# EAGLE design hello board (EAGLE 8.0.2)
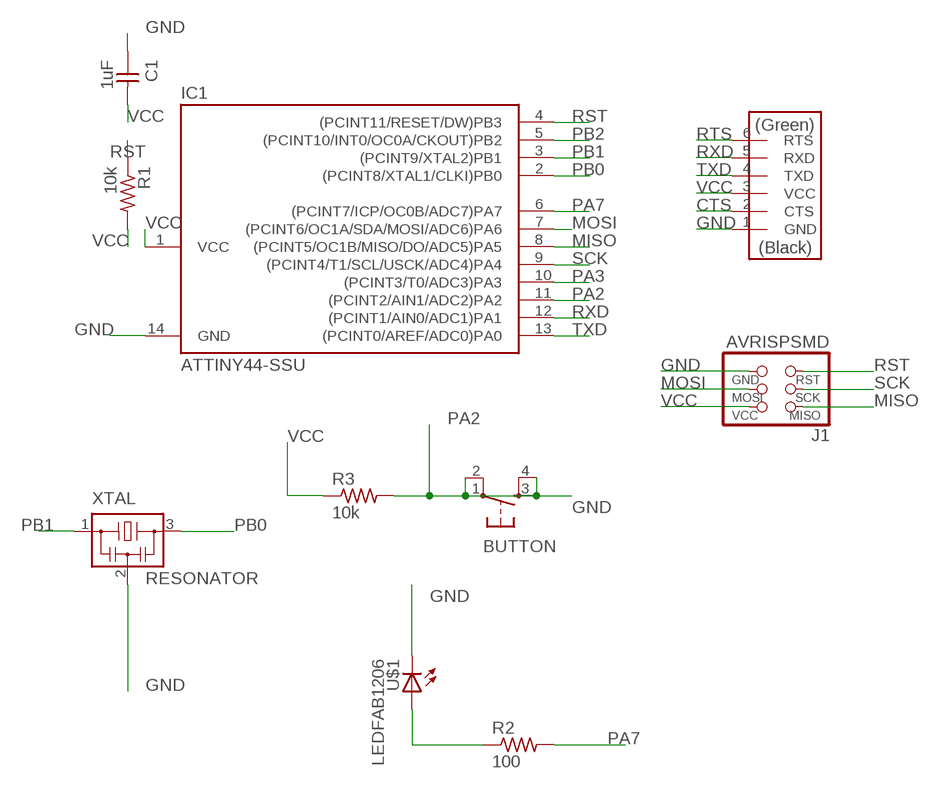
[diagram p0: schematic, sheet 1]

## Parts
BUTTON  6MM_SWITCH6MM_SWITCH  [6MM_SWITCH]
C1  1uF  CAP-UNPOLARIZEDFAB  [C1206FAB]
IC1  ATTINY44-SSU  [SOIC14]
J1  AVRISPSMD  [2X03SMD]
R1  10k  RES-US1206W  [R1206W]
R2  100  RES-US1206FAB  [R1206FAB]
R3  10k  RES-US1206FAB  [R1206FAB]
U$1  LEDFAB1206  [LED1206FAB]
U$2  FTDI-SMD-HEADER  [1X06SMD]
XTAL  RESONATOR  [EFOBM]

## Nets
CTS: U$2.2(CTS)
GND: BUTTON.1(P) BUTTON.2(P1) C1.1 IC1.14(GND) J1.6(GND) U$1.2(C) U$2.1(GND) XTAL.2
MISO: IC1.8((PCINT5/OC1B/MISO/DO/ADC5)PA5) J1.1(MISO)
MOSI: IC1.7((PCINT6/OC1A/SDA/MOSI/ADC6)PA6) J1.4(MOSI)
N$1: R2.1 U$1.1(A)
PA2: BUTTON.3(S) BUTTON.4(S1) IC1.11((PCINT2/AIN1/ADC2)PA2) R3.2
PA3: IC1.10((PCINT3/T0/ADC3)PA3)
PA7: IC1.6((PCINT7/ICP/OC0B/ADC7)PA7) R2.2
PB0: IC1.2((PCINT8/XTAL1/CLKI)PB0) XTAL.3
PB1: IC1.3((PCINT9/XTAL2)PB1) XTAL.1
PB2: IC1.5((PCINT10/INT0/OC0A/CKOUT)PB2)
RST: IC1.4((PCINT11/RESET/DW)PB3) J1.5(RST) R1.1
RTS: U$2.6(RTS)
RXD: IC1.12((PCINT1/AIN0/ADC1)PA1) U$2.5(RXD)
SCK: IC1.9((PCINT4/T1/SCL/USCK/ADC4)PA4) J1.3(SCK)
TXD: IC1.13((PCINT0/AREF/ADC0)PA0) U$2.4(TXD)
VCC: C1.2 IC1.1(VCC) J1.2(VCC) R1.2 R3.1 U$2.3(VCC)

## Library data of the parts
BUTTON = fab:6MM_SWITCH: OMRON SWITCH
C1 = fab:CAP-UNPOLARIZED
IC1 = fab:ATTINY44
J1 = fab:AVRISP
R1-R3 = fab:RES-US: Resistor (US Symbol)
U$1 = fab:LED: LED
U$2 = fab:FTDI-SMD-HEADER
XTAL = fab:RESONATOR

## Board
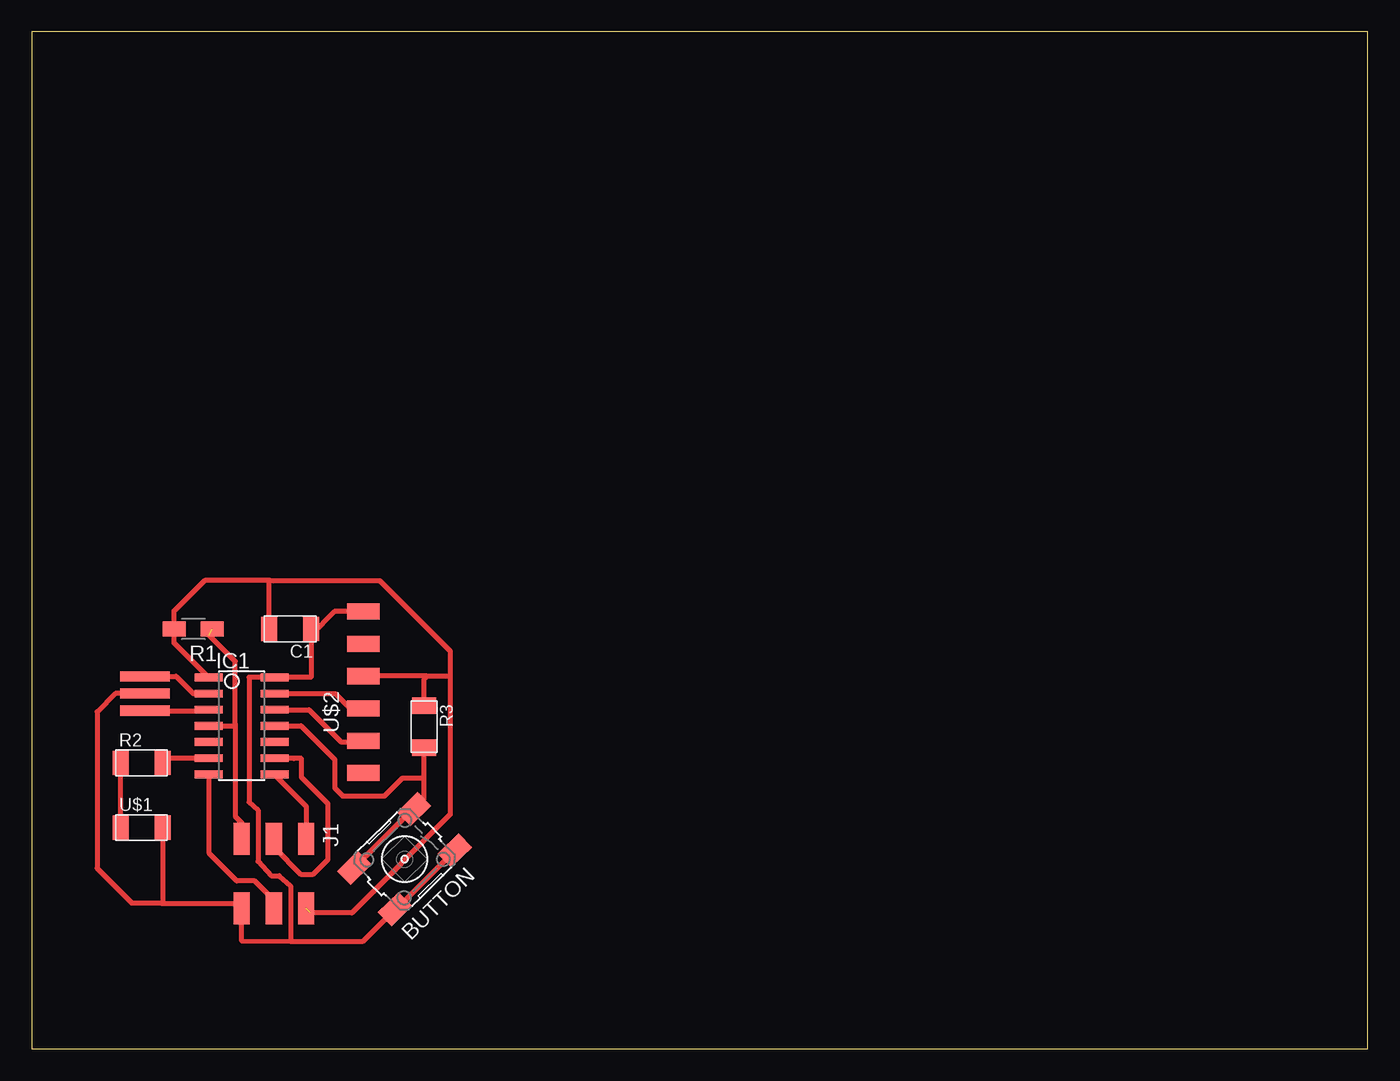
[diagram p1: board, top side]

Size 105.08 x 80 mm. Coordinates in mm from the lower left corner, seen from the top.
Outline: 0,0 105.08,0 105.08,80 0,80 0,0
Copper layers (1*16): Top 0.035mm / dielectric 1.5mm / Bottom 0.035mm
Design rules "default *": minimum track width 10mil, minimum drill 24mil, track to track 16mil, track to pad 16mil, pad to pad 16mil, via to via 16mil, smd to smd 16mil, copper to edge 40mil, drill to drill 8mil, minimum pad ring 10mil, minimum via ring 8mil, stop-mask expansion 4mil, vias tented up to drill 0mil, thermal gap 10mil

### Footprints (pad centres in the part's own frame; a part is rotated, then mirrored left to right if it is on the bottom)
6MM_SWITCH = smd 2.286 x 1.524: 1 -3.302,2.286; 2 3.302,2.286; 3 -3.302,-2.286; 4 3.302,-2.286
C1206FAB = smd 1.27 x 1.905: 1 -1.651,0; 2 1.651,0
SOIC14 = smd 0.61 x 2.21: 1 -3.81,-2.603; 2 -2.54,-2.603; 3 -1.27,-2.603; 4 0,-2.603; 5 1.27,-2.603; 6 2.54,-2.603; 7 3.81,-2.603; 8 3.81,2.603; 9 2.54,2.603; 10 1.27,2.603; 11 0,2.603; 12 -1.27,2.603; 13 -2.54,2.603; 14 -3.81,2.603
2X03SMD = smd 2.54 x 1.27: 1 -2.54,2.54; 2 2.92,2.54; 3 -2.54,0; 4 2.92,0; 5 -2.54,-2.54; 6 2.92,-2.54
R1206W = smd 1.8 x 1.2: 1 -1.499,0; 2 1.499,0
R1206FAB = smd 1.27 x 1.905: 1 -1.651,0; 2 1.651,0
LED1206FAB = smd 1.27 x 1.905: 1 -1.651,0; 2 1.651,0
1X06SMD = smd 2.54 x 1.27: 1 0,6.35; 2 0,3.81; 3 0,1.27; 4 0,-1.27; 5 0,-3.81; 6 0,-6.35
EFOBM = smd 0.8 x 3.9: 1 -1.35,0; 2 0,0; 3 1.35,0

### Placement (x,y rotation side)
BUTTON  29.32,14.92 224.5 top
C1  20.32,33.02 180 top
IC1  16.51,25.4 270 top
J1  19.05,13.97 270 top
R1  12.7,33.02 180 top
R2  8.64,22.48 0 top
R3  30.86,25.33 270 top
U$1  8.64,17.4 0 top
U$2  26.08,28.04 0 top
XTAL  8.89,27.94 90 top

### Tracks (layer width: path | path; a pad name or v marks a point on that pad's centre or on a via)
GND
  Top 0.406: 21.59,33.02 C1.1 21.97,32.56 | J1.6 16.51,11.43 | XTAL.2 6.57,27.94 5.13,26.5 5.13,14.2 7.88,11.45 10.18,11.45 | 10.18,11.45 16.11,11.45 J1.6 | U$1.2 10.29,11.56 10.18,11.45 | 20.32,8.46 16.52,8.48 J1.6 | 26.06,34.4 U$2.1 23.8,34.39 21.97,32.56 | 19.16,29.16 IC1.14 | 21.97,32.56 21.97,29.21 IC1.14 | IC1.14 17.08,29.21 17.08,19.42 17.8,18.77 17.8,14.73 18.84,13.62 19.46,13.62 20.34,12.82 20.34,8.52 20.32,8.46 | 20.32,8.46 26.06,8.46 BUTTON.2 28.65,10.97 BUTTON.1
MISO
  Top 0.406: IC1.8 19.11,21.53 21.59,19.05 J1.1
MOSI
  Top 0.406: 13.97,21.59 IC1.7 13.97,21.53 13.97,15.37 16.13,13.21 17.53,13.21 19.05,11.68 J1.4
N$1
  Top 0.406: U$1.1 R2.1
PA2
  Top 0.406: IC1.11 21.17,25.4 23.83,22.75 23.83,20.5 24.45,19.89 27.74,19.89 29.16,21.3 30.81,21.3 | 30.81,21.3 30.84,21.34 30.84,23.66 R3.2 | 30.81,21.3 30.81,19.6 BUTTON.3 29.99,18.86 BUTTON.4
PA7
  Top 0.406: IC1.6 10.67,22.86 R2.2
PB0
  Top 0.406: XTAL.3 11.35,29.29 12.7,27.94 IC1.2
PB1
  Top 0.406: XTAL.1 13.83,26.59 IC1.3
RST  (1 unrouted)
  Top 0.406: J1.5 16.51,17.78 16,18.29 16,25.53 | 16,25.53 16,30.48 13.97,32.51 | IC1.4 15.88,25.4 16,25.53
RXD
  Top 0.406: IC1.12 21.8,26.67 24.33,24.15 25.99,24.15 U$2.5
SCK
  Top 0.406: IC1.9 20.59,22.86 20.62,22.83 21.21,22.83 21.21,21.36 23.3,19.28 23.3,14.88 22.14,13.73 21.15,13.73 19.05,15.83 J1.3
TXD
  Top 0.406: IC1.13 23.87,27.94 25.03,26.77 U$2.4
VCC  (1 unrouted)
  Top 0.406: IC1.1 11.2,31.92 R1.2 11.2,34.45 13.59,36.83 18.78,36.83 | 32.91,29.22 32.91,31.28 27.37,36.83 18.78,36.83 | J1.2 21.7,10.95 | 31.09,29.31 U$2.3 | 31.09,29.31 32.83,29.31 32.91,29.22 | R3.1 30.86,29.08 31.09,29.31 | C1.2 18.67,36.72 18.78,36.83 | 21.95,10.69 25.19,10.69 32.91,18.42 32.91,29.22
